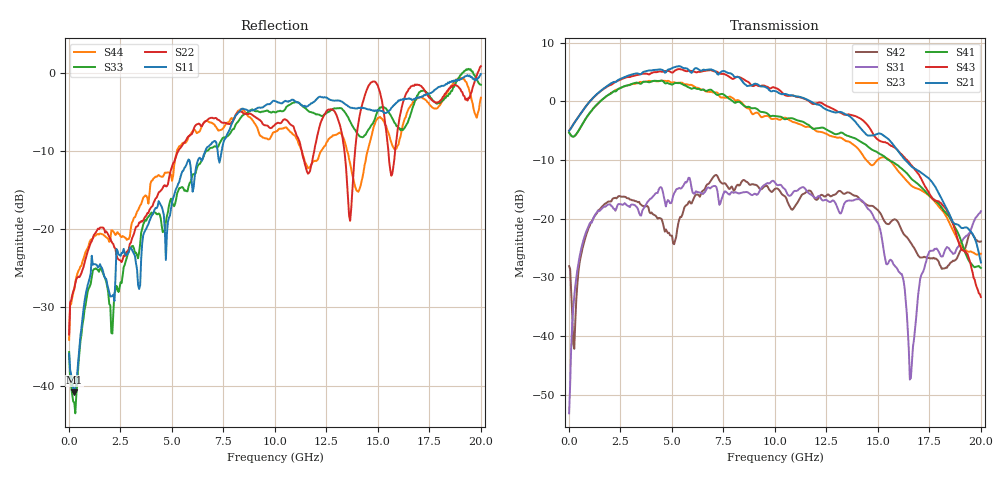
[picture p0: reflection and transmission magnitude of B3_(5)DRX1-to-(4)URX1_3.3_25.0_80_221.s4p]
!Agilent Technologies,N5225A,MY51451112,A.09.50.13
!Agilent N5225A: A.09.50.13
!Date: Sunday, March 12, 2017 05:23:03
!Correction: S11(Full 4 Port(1,2,3,4))
!S12(Full 4 Port(1,2,3,4))
!S13(Full 4 Port(1,2,3,4))
!S14(Full 4 Port(1,2,3,4))
!S21(Full 4 Port(1,2,3,4))
!S22(Full 4 Port(1,2,3,4))
!S23(Full 4 Port(1,2,3,4))
!S24(Full 4 Port(1,2,3,4))
!S31(Full 4 Port(1,2,3,4))
!S32(Full 4 Port(1,2,3,4))
!S33(Full 4 Port(1,2,3,4))
!S34(Full 4 Port(1,2,3,4))
!S41(Full 4 Port(1,2,3,4))
!S42(Full 4 Port(1,2,3,4))
!S43(Full 4 Port(1,2,3,4))
!S44(Full 4 Port(1,2,3,4))
!S4P File: Measurements: <S11,S12,S13,S14>,
!<S21,S22,S23,S24>,
!<S31,S32,S33,S34>,
!<S41,S42,S43,S44>:
# Hz S  dB  R 50
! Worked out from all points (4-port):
!   401 points, 10 MHz to 20 GHz, reference 50 ohm
!   strongest paths, dB at 10 MHz, 5.008 GHz, 10.01 GHz, 15 GHz, 20 GHz:
!     S21: -5.0, 5.7, 1.8, -5.5, -27.5
!     S43: -5.0, 4.9, 2.3, -6.5, -33.3
!     S41: -5.3, 2.9, -2.5, -8.8, -28.4
!     S23: -5.3, 3.2, -2.9, -9.9, -26.0
!     S31: -53.2, -17.0, -13.9, -20.8, -18.7
!     S42: -28.1, -22.9, -14.9, -18.5, -23.9
!   lowest |S11| = -40.8 dB at 259.9 MHz (marker M1), VSWR 1.02, Z = 50.3 - j0.869 ohm
!   |S11| at or under -10 dB: start of sweep to 6.626 GHz; 7.219 GHz to 7.416 GHz (197.2 MHz wide, 2.69 % of centre)
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1e7  -35.93 -38.7  -66.57 138.8  -52.59 11.9  -66.66 130.6
     -5.01 1.9  -33.46 39.7  -5.33 -179.5  -28.01 38.0
     -53.18 26.9  -63.91 71.8  -35.72 -46.4  -64.94 150.7
     -5.33 -179.5  -28.08 38.3  -5.00 2.1  -34.14 44.5
2.59875e8  -40.85 -72.2  -49.93 56.9  -33.11 94.9  -50.48 52.7
           -3.67 6.2  -27.61 -131.9  -5.93 -179.1  -41.86 -162.1
           -33.22 95.1  -49.77 54.4  -42.13 -78.5  -50.46 53.7
           -5.94 -179.9  -42.18 -170.5  -3.66 5.4  -27.65 -137.7
2.90855e9  -22.99 148.7  -40.89 -36.4  -17.65 54.1  -39.12 -50.5
           4.44 -92.2  -22.54 158.3  2.81 80.5  -16.40 40.1
           -17.89 53.4  -39.89 -32.3  -22.61 121.8  -37.94 -44.0
           2.76 70.6  -16.52 40.6  4.15 -100.2  -21.25 140.9
5.0075e9  -16.53 93.6  -44.21 -11.3  -16.29 28.0  -38.04 -35.5
          5.67 170.9  -11.98 148.5  3.20 -25.0  -24.88 38.3
          -16.96 26.8  -38.15 1.5  -16.56 102.4  -32.66 -16.9
          2.87 -40.4  -22.90 37.3  4.89 158.5  -13.82 117.4
7.956025e9  -6.25 41.5  -32.73 -101.8  -16.51 7.5  -31.97 -122.0
            4.53 23.1  -6.17 88.5  0.58 -164.1  -14.42 50.7
            -15.52 6.1  -29.93 -102.2  -7.21 64.9  -30.66 -132.8
            0.05 170.8  -14.88 48.1  3.82 11.8  -5.95 42.8
1.155422e10  -4.31 -6.1  -37.47 -117.9  -14.75 -22.4  -40.04 -137.1
             0.32 -132.7  -12.61 85.3  -4.32 41.9  -15.37 37.0
             -15.27 -23.5  -33.56 -123.1  -4.73 10.4  -34.11 -152.2
             -3.87 4.1  -15.36 42.5  0.27 -157.7  -11.88 25.4
2e10  -0.17 -114.2  -32.95 63.2  -18.74 121.2  -35.49 21.4
      -27.46 -163.3  0.84 17.1  -25.96 21.4  -23.89 101.9
      -18.72 121.2  -33.98 40.3  -1.53 -87.7  -35.25 -7.5
      -28.40 -27.0  -23.88 102.8  -33.35 166.9  -3.18 -136.7
